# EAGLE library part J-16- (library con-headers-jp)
HEADER JACK PINS
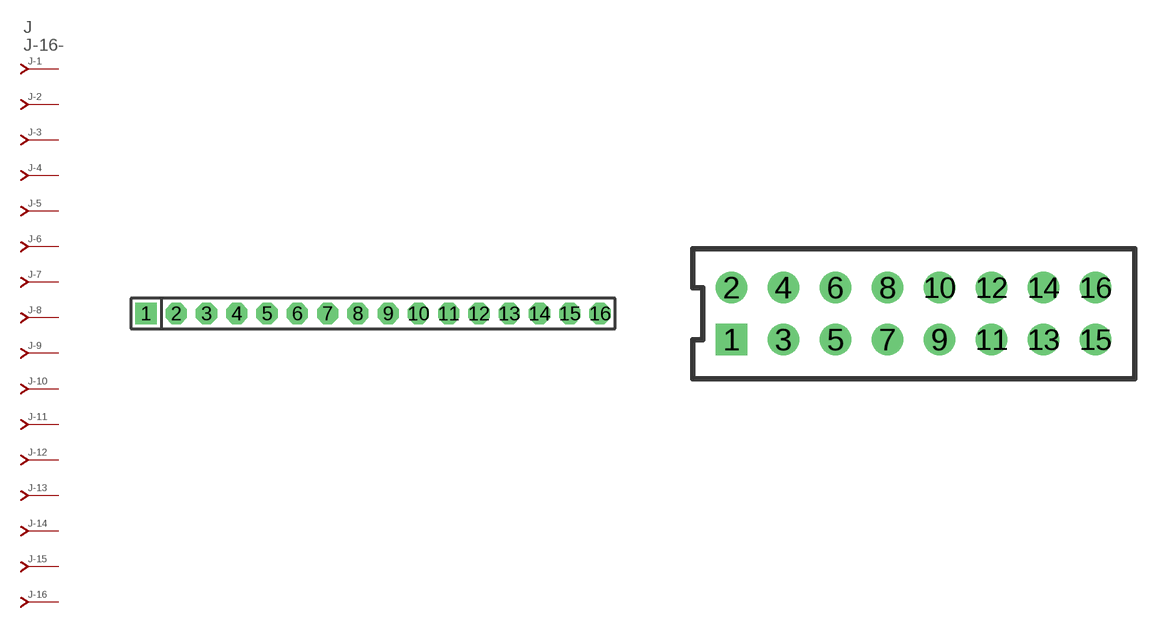
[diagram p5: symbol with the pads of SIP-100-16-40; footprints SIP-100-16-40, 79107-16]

Designator prefix J; gates -2=J-N -3=J-N -4=J-N -5=J-N -6=J-N -7=J-N -8=J-N -9=J-N -10=J-N -11=J-N -12=J-N -13=J-N -14=J-N -15=J-N -16=J-N -1=J-NV

## J-16-SIP-100-40  [SIP-100-16-40]
1  -1:J  pas
2  -2:J  pas
3  -3:J  pas
4  -4:J  pas
5  -5:J  pas
6  -6:J  pas
7  -7:J  pas
8  -8:J  pas
9  -9:J  pas
10  -10:J  pas
11  -11:J  pas
12  -12:J  pas
13  -13:J  pas
14  -14:J  pas
15  -15:J  pas
16  -16:J  pas

## J-16-79107  [79107-16]
Pads as for SIP-100-16-40

## J-16-79109  [79109-16]
Pads as for SIP-100-16-40

## J-16-87264  [87264-16]
Pads as for SIP-100-16-40

## J-16-87368  [87368-16]
Pads as for SIP-100-16-40

## J-16-535512  [535512-16]
Pads as for SIP-100-16-40

## J-16-87340  [87340-16]
Pads as for SIP-100-16-40

## J-16-100-2X08  [DIL-100-2X08]
Pads as for SIP-100-16-40

## J-16-100-2X08_M  [DIL-100-2X08_M]
Pads as for SIP-100-16-40

## J-16-2MM-2X08  [DIL-2MM-2X08]
Pads as for SIP-100-16-40

## J-16-2MM-2X08_M  [DIL-2MM-2X08_M]
Pads as for SIP-100-16-40

## J-16-SIP-100-32  [SIP-100-16-32]
Pads as for SIP-100-16-40

## J-16-SIP-100-40Y  [SIP-100-16-40Y]
Pads as for SIP-100-16-40

## J-16-SIP-100-32Y  [SIP-100-16-32Y]
Pads as for SIP-100-16-40

## J-16-71991  [71991-16]
Pads as for SIP-100-16-40

## J-16-KK-4455-B16  [KK-4455-B16]
Pads as for SIP-100-16-40

## J-16-KK-4455-A16  [KK-4455-A16]
Pads as for SIP-100-16-40

## J-16-KK-4455-C16  [KK-4455-C16]
Pads as for SIP-100-16-40

## Footprint SIP-100-16-40 (pad centres in mm)
SIP Header - 0.1", 40 mil drill
drill 1.016 pad 1.778 square: 1 -19.05,0
drill 1.016 pad 1.778 octagon: 2 -16.51,0; 3 -13.97,0; 4 -11.43,0; 5 -8.89,0; 6 -6.35,0; 7 -3.81,0; 8 -1.27,0; 9 1.27,0; 10 3.81,0; 11 6.35,0; 12 8.89,0; 13 11.43,0; 14 13.97,0; 15 16.51,0; 16 19.05,0

## Footprint 79107-16 (pad centres in mm)
Molex Board-To-Board Receptacal 2.00mm (.079") Pitch Milli-Grid Header, Vertical, Through-Hole Mates with: 87759, 87762, 87758, 87760
drill 0.711 square: 1 -7,-1
drill 0.711: 2 -7,1; 3 -5,-1; 4 -5,1; 5 -3,-1; 6 -3,1; 7 -1,-1; 8 -1,1; 9 1,-1; 10 1,1; 11 3,-1; 12 3,1; 13 5,-1; 14 5,1; 15 7,-1; 16 7,1

## Footprint 79109-16 (pad centres in mm)
Molex Board-to-Board Receptacal 2.00mm (.079") Pitch Milli-Grid Header, Vertical, Top/Bottom Entry Mates with: 87758, 87759, 87760, 87831, 87832, 87833
smd 1.12 x 1.83: 1 -7,-2.65; 2 -7,2.65; 3 -5,-2.65; 4 -5,2.65; 5 -3,-2.65; 6 -3,2.65; 7 -1,-2.65; 8 -1,2.65; 9 1,-2.65; 10 1,2.65; 11 3,-2.65; 12 3,2.65; 13 5,-2.65; 14 5,2.65; 15 7,-2.65; 16 7,2.65
hole 0.914 at -6,0
hole 0.914 at -7,1
hole 0.914 at -7,-1
hole 0.914 at -5,-1
hole 0.914 at -5,1
hole 0.914 at -3,-1
hole 0.914 at -3,1
hole 0.914 at 6,0
hole 0.914 at -1,1
hole 0.914 at -1,-1
hole 0.914 at 1,1
hole 0.914 at 1,-1
hole 0.914 at 3,1
hole 0.914 at 3,-1
hole 0.914 at 5,1
hole 0.914 at 5,-1
hole 0.914 at 7,-1
hole 0.914 at 7,1

## Footprint 87264-16 (pad centres in mm)
Molex Board-To-Board Receptacal 2.00mm (.079") Pitch Milli-Grid Header, Side Entry Mates with 2mm(.079") Mill-Grid Header
drill 0.914 square: 1 -7,-2.25
drill 0.914: 2 -7,2.25; 3 -5,-2.25; 4 -5,2.25; 5 -3,-2.25; 6 -3,2.25; 7 -1,-2.25; 8 -1,2.25; 9 1,-2.25; 10 1,2.25; 11 3,-2.25; 12 3,2.25; 13 5,-2.25; 14 5,2.25; 15 7,-2.25; 16 7,2.25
